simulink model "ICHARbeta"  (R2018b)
settings: Solver=ode5  StartTime=0.0  StopTime=20  FixedStep=0.01  RelTol=1e-3  AbsTol=1e-6
undefined symbols (not defined in the file or in its folder): Crane3D_RangeBit, Crane3D_ScaleCoeff, rtdac4pciebaseaddress
libraries: simulink x1

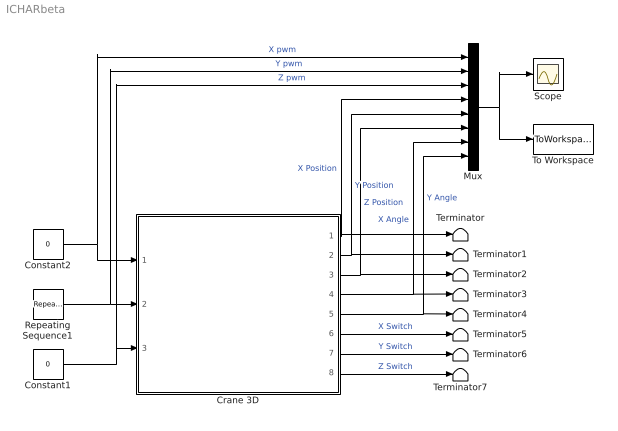
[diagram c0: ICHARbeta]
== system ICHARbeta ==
  Constant1 : Constant  Value=0
  Constant2 : Constant  Value=0
  Crane 3D : Subsystem  mask{BaseAddress=rtdac4pciebaseaddress, T0=0.01}
      mask prompts: BaseAddress "Base Address:"; T0 "Sampling Period:"
  Mux : Mux  Inputs=8
  Repeating Sequence1 : simulink/Sources/Repeating Sequence  rep_seq_t=[0 1.99 2 2.99 3 5 20]  rep_seq_y=[0 0 1 1 0 0 0]
  Scope : Scope
  Terminator{,1..7} (8 alike) : Terminator
  To Workspace : ToWorkspace  VariableName=simout  SaveFormat=Timeseries  SampleTime=-1
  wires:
  Crane 3D/6(X Switch) -> Terminator5/1  "X Switch"
  Crane 3D/7(Y Switch) -> Terminator6/1  "Y Switch"
  Crane 3D/8(Z Switch) -> Terminator7/1  "Z Switch"
  Crane 3D/1(X Position) -> Mux/4, Terminator/1  "X Position"
  Crane 3D/2(Y Position) -> Mux/5, Terminator1/1  "Y Position"
  Crane 3D/3(Z Position) -> Mux/6, Terminator2/1  "Z Position"
  Mux/1 -> To Workspace/1, Scope/1
  Crane 3D/4(X Angle) -> Mux/7, Terminator3/1  "X Angle"
  Crane 3D/5(Y Angle) -> Mux/8, Terminator4/1  "Y Angle"
  Constant2/1 -> Mux/1, Crane 3D/1(X PWM)  "X pwm"
  Repeating Sequence1/1 -> Mux/2, Crane 3D/2(Y PWM)  "Y pwm"
  Constant1/1 -> Mux/3, Crane 3D/3(Z PWM)  "Z pwm"

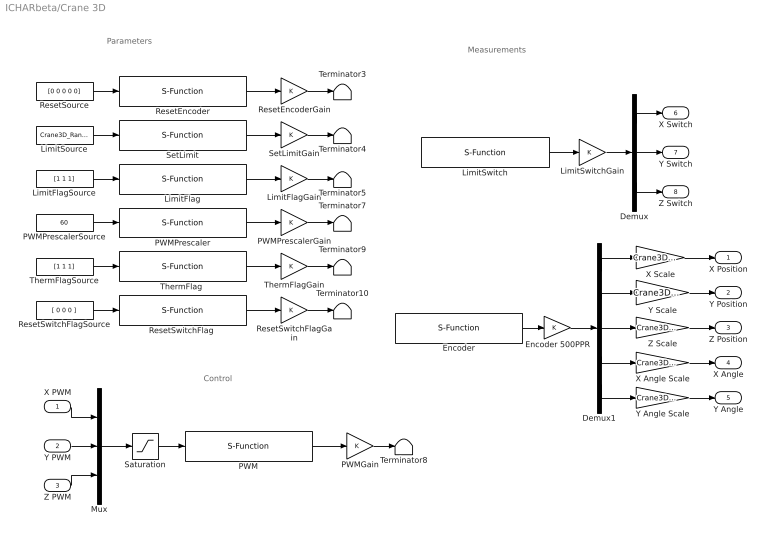
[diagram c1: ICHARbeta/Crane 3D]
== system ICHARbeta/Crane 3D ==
  note: Parameters
  note: Control
  note: Measurements
  X PWM : Inport
  Y PWM : Inport  Port=2
  Z PWM : Inport  Port=3
  Demux : Demux  Outputs=3
  Demux1 : Demux  Outputs=5
  Encoder : S-Function  FunctionName=Crane3D_Encoder  Parameters=BaseAddress, T0  SFunctionDeploymentMode=off  EnableBusSupport=off
  Encoder 500PPR : Gain
  LimitFlag : S-Function  FunctionName=Crane3D_LimitFlag  Parameters=BaseAddress, T0  SFunctionDeploymentMode=off  EnableBusSupport=off
  LimitFlagGain : Gain
  LimitFlagSource : Constant  Value=[1 1 1]
  LimitSource : Constant  Value=Crane3D_RangeBit
  LimitSwitch : S-Function  FunctionName=Crane3D_Switch  Parameters=BaseAddress, T0  SFunctionDeploymentMode=off  EnableBusSupport=off
  LimitSwitchGain : Gain
  Mux : Mux  Inputs=3
  PWM : S-Function  FunctionName=Crane3D_PWM  Parameters=BaseAddress, T0  SFunctionDeploymentMode=off  EnableBusSupport=off
  PWMGain : Gain
  PWMPrescaler : S-Function  FunctionName=Crane3D_PWMPrescaler  Parameters=BaseAddress, T0  SFunctionDeploymentMode=off  EnableBusSupport=off
  PWMPrescalerGain : Gain
  PWMPrescalerSource : Constant  Value=60
  ResetEncoder : S-Function  FunctionName=Crane3D_ResetEncoder  Parameters=BaseAddress, T0  SFunctionDeploymentMode=off  EnableBusSupport=off
  ResetEncoderGain : Gain
  ResetSource : Constant  Value=[0 0 0 0 0]
  "ResetSwitchFlag " : S-Function  FunctionName=Crane3D_ResetSwitchFlag  Parameters=BaseAddress, T0  SFunctionDeploymentMode=off  EnableBusSupport=off
  ResetSwitchFlagGain : Gain
  ResetSwitchFlagSource : Constant  Value=[ 0 0 0 ]
  Saturation : Saturate  UpperLimit=1  LowerLimit=-1
  SetLimit : S-Function  FunctionName=Crane3D_SetLimit  Parameters=BaseAddress, T0  SFunctionDeploymentMode=off  EnableBusSupport=off
  SetLimitGain : Gain
  Terminator{3..5,7..10} (7 alike) : Terminator
  "ThermFlag " : S-Function  FunctionName=Crane3D_ThermFlag  Parameters=BaseAddress, T0  SFunctionDeploymentMode=off  EnableBusSupport=off
  ThermFlagGain : Gain
  ThermFlagSource : Constant  Value=[1 1 1]
  X Angle Scale : Gain  Gain=Crane3D_ScaleCoeff( 4 )
  X Scale : Gain  Gain=Crane3D_ScaleCoeff( 1 )
  Y Angle Scale : Gain  Gain=Crane3D_ScaleCoeff( 5 )
  Y Scale : Gain  Gain=Crane3D_ScaleCoeff( 2 )
  Z Scale : Gain  Gain=Crane3D_ScaleCoeff( 3 )
  X Position : Outport  InitialOutput=0
  Y Position : Outport  Port=2  InitialOutput=0
  Z Position : Outport  Port=3  InitialOutput=0
  X Angle : Outport  Port=4  InitialOutput=0
  Y Angle : Outport  Port=5  InitialOutput=0
  X Switch : Outport  Port=6  InitialOutput=0
  Y Switch : Outport  Port=7  InitialOutput=0
  Z Switch : Outport  Port=8  InitialOutput=0
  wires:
  Encoder 500PPR/1 -> Demux1/1
  Encoder/1 -> Encoder 500PPR/1
  Saturation/1 -> PWM/1
  Mux/1 -> Saturation/1
  PWM/1 -> PWMGain/1
  PWMGain/1 -> Terminator8/1
  ResetEncoder/1 -> ResetEncoderGain/1
  SetLimit/1 -> SetLimitGain/1
  LimitFlag/1 -> LimitFlagGain/1
  PWMPrescaler/1 -> PWMPrescalerGain/1
  "ThermFlag "/1 -> ThermFlagGain/1
  "ResetSwitchFlag "/1 -> ResetSwitchFlagGain/1
  ResetSource/1 -> ResetEncoder/1
  LimitSource/1 -> SetLimit/1
  LimitFlagSource/1 -> LimitFlag/1
  PWMPrescalerSource/1 -> PWMPrescaler/1
  ThermFlagSource/1 -> "ThermFlag "/1
  ResetSwitchFlagSource/1 -> "ResetSwitchFlag "/1
  ResetEncoderGain/1 -> Terminator3/1
  SetLimitGain/1 -> Terminator4/1
  LimitFlagGain/1 -> Terminator5/1
  PWMPrescalerGain/1 -> Terminator7/1
  ThermFlagGain/1 -> Terminator9/1
  ResetSwitchFlagGain/1 -> Terminator10/1
  Z PWM/1 -> Mux/3
  Y PWM/1 -> Mux/2
  X PWM/1 -> Mux/1
  LimitSwitch/1 -> LimitSwitchGain/1
  LimitSwitchGain/1 -> Demux/1
  Demux/1 -> X Switch/1
  Demux/2 -> Y Switch/1
  Demux/3 -> Z Switch/1
  Z Scale/1 -> Z Position/1
  X Scale/1 -> X Position/1
  Y Scale/1 -> Y Position/1
  Y Angle Scale/1 -> Y Angle/1
  X Angle Scale/1 -> X Angle/1
  Demux1/5 -> Y Angle Scale/1
  Demux1/4 -> X Angle Scale/1
  Demux1/3 -> Z Scale/1
  Demux1/2 -> Y Scale/1
  Demux1/1 -> X Scale/1
